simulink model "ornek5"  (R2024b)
settings: Solver=VariableStepAuto  StartTime=0.0  StopTime=10.0  RelTol=1e-3

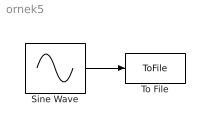
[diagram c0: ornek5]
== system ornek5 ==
  Sine Wave : Sin  Frequency=100*pi  SampleTime=0.02/32
  To File : ToFile  Filename=kayit.mat  MatrixName=v
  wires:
  Sine Wave/1 -> To File/1
